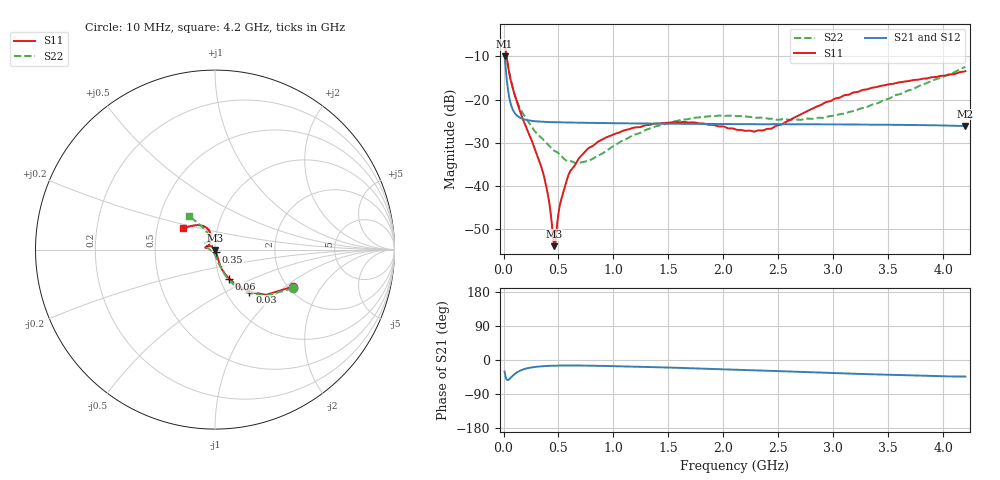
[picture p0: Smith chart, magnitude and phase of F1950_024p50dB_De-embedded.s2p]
! Integrated Device Technology
! Corporate Headquarters
! 6024 Silver Creek Valley Road
! San Jose, CA 95138  USA
! Phone:  1-408-284-8200
! Toll Free:  1-800-223-1366
! Webpage:  http://www.idt.com/
! Timing and RF Division
! 515 Groton Road, Suite 102
! Westford, MA 01886-6024
! Device:  F1950
! Description: 7-bit 0.25 dB Digital Step Attenuator
! Frequency:  150.0 -  4000.00 MHz
! Package:  4x4 mm Thin QFN Plastic Package: 24 pin
! Ports:  2 RF, 12 DC
!  Pin  1  = D0
!  Pin  2  = VDD
!  Pin  3  = Vmode
!  Pin  4  = GND
!  Pin  5  = RF1  =  Port 1
!  Pin  6  = GND
!  Pin  7  = GND
!  Pin  8  = GND
!  Pin  9  = GND
!  Pin 10  = GND
!  Pin 11  = GND
!  Pin 12  = GND
!  Pin 13  = GND
!  Pin 14  = RF2  =  Port 2
!  Pin 15  = GND
!  Pin 16  = LE
!  Pin 17  = CLK
!  Pin 18  = DATE
!  Pin 19  = D6
!  Pin 20  = D5
!  Pin 21  = D4
!  Pin 22  = D3
!  Pin 23  = D2
!  Pin 24  = D1
! State:  98
! Atten State:  24.50 dB
! Voltage:  +5.00 Volts
! Current:  Not Measured mA
! Data:  The device was measured on a the F195X evaluation board which has
!  individual transmission lines to the RF pins.  Data was collected
!  using a calibrated network analyzer.  The evaluation board was
!  de-embedded using a TRL calibration technique.
!  The reference plane is the edge of the package pin.
! Misc:  Board 2019
!  Action Tracker AT0250
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# GHz S dB R 50
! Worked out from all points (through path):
!   420 points, 10 MHz to 4.2 GHz, reference 50 ohm
!   highest |S21| = -9.98 dB at 10 MHz (marker M1); lowest = -26.1 dB at 4.2 GHz (marker M2)
!   group delay of S21, straight-line fit = 18 ps
!   lowest |S11| = -54.0 dB at 460 MHz (marker M3), VSWR 1.00, Z = 49.8 - j0.132 ohm
!   |S11| at or under -10 dB: 28.17 MHz to end of sweep
!   |S22| runs from -34.8 to -6.3 dB; largest |S21 - S12| = 0.0001
!   S11 on the Smith chart (normalised r, x): 10 MHz: 2.12, -1.14; 30 MHz: 1.28, -0.66; 60 MHz: 1.11, -0.37; 350 MHz: 1.01, -0.03; 4.2 GHz: 0.68, +0.17
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0.01  -6.37 -25.4  -9.98 -30.8  -9.98 -30.8  -6.30 -26.4
0.03  -10.36 -50.7  -15.45 -52.1  -15.45 -52.1  -10.29 -52.2
0.06  -14.86 -63.9  -20.44 -48.5  -20.44 -48.5  -14.65 -65.4
0.1  -18.76 -70.6  -23.04 -37.4  -23.04 -37.3  -18.74 -71.0
0.15  -22.71 -72.6  -24.19 -28.3  -24.19 -28.3  -21.99 -75.2
0.35  -36.12 -71.1  -25.13 -16.5  -25.13 -16.5  -28.97 -85.7
0.4  -41.55 -76.0  -25.19 -15.6  -25.19 -15.6  -30.32 -87.7
0.45  -51.63 -111.0  -25.24 -15.1  -25.24 -15.1  -31.63 -93.9
0.46  -53.96 -138.8  -25.24 -15.0  -25.24 -15.0  -31.81 -95.6
0.48  -50.90 164.3  -25.26 -14.9  -25.26 -14.9  -32.10 -98.5
0.52  -43.61 144.5  -25.28 -14.6  -25.28 -14.6  -32.88 -101.9
0.58  -38.30 137.6  -25.31 -14.5  -25.31 -14.5  -34.18 -113.9
0.71  -32.95 139.3  -25.37 -14.7  -25.37 -14.7  -34.52 -138.5
0.99  -28.17 148.3  -25.47 -16.1  -25.47 -16.2  -30.94 -178.5
1.41  -25.53 163.8  -25.57 -19.3  -25.57 -19.3  -26.02 161.7
1.73  -25.28 169.1  -25.62 -21.9  -25.61 -21.9  -24.23 153.2
2.11  -26.91 159.2  -25.67 -25.7  -25.67 -25.7  -23.82 143.5
2.43  -26.74 128.0  -25.70 -28.5  -25.70 -28.5  -24.43 133.0
2.81  -22.12 106.4  -25.73 -32.4  -25.73 -32.4  -24.45 117.8
3.1  -18.99 107.8  -25.76 -35.3  -25.76 -35.4  -23.22 112.8
3.51  -16.43 118.1  -25.82 -39.2  -25.82 -39.2  -19.73 114.4
4.2  -13.41 145.9  -26.13 -43.7  -26.13 -43.8  -12.43 127.7
